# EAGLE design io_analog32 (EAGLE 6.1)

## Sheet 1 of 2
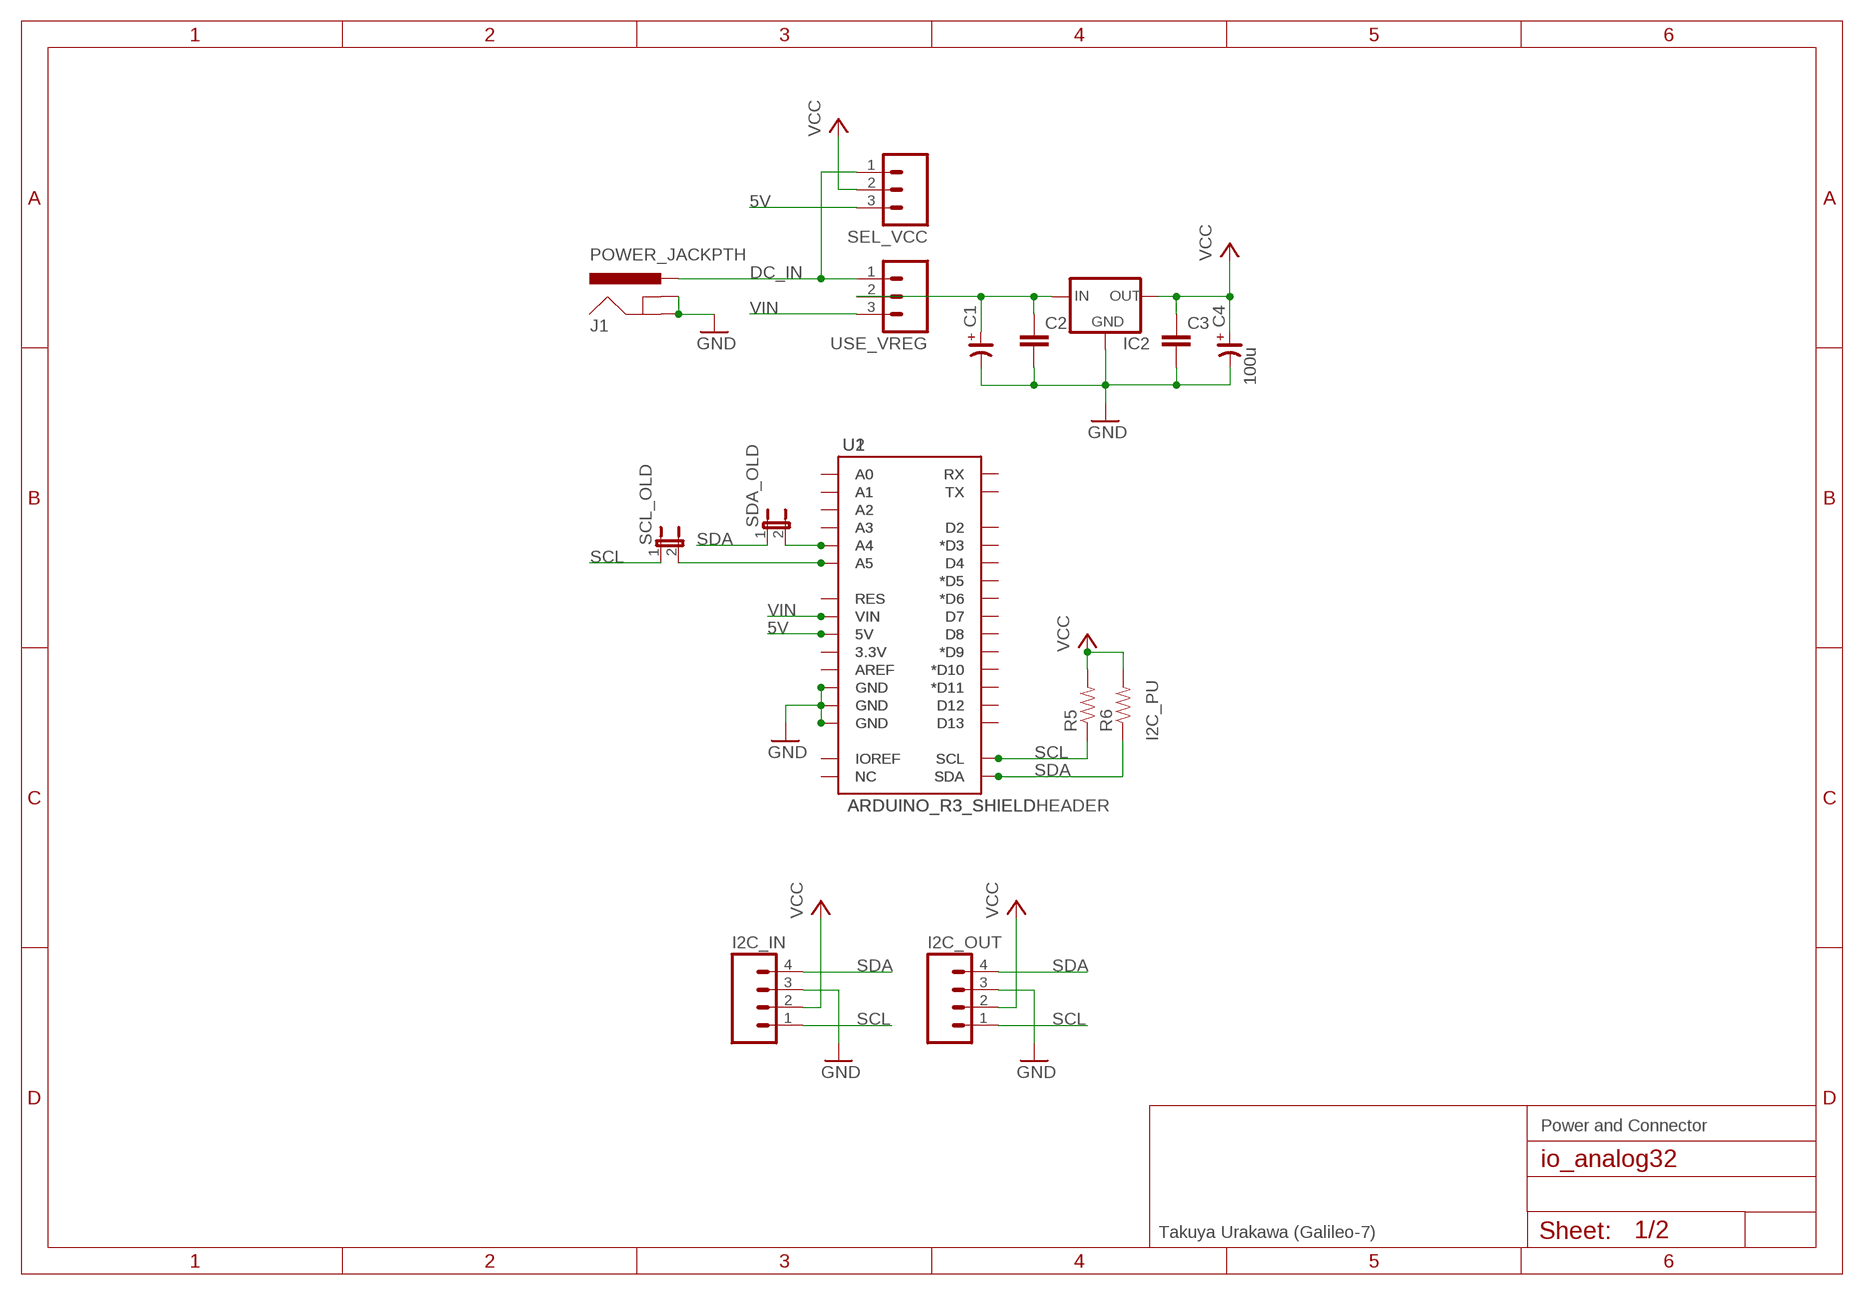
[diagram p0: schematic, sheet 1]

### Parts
C1  CP_E-025X065  [CE-025X065]
C2  CAPPTH1  [CAP-PTH-5MM]
C3  CAPPTH1  [CAP-PTH-5MM]
C4  100u  CP_E-025X065  [CE-025X065]
I2C_IN  M04PTH  [1X04]
I2C_OUT  M04PTH  [1X04]
IC2  V_REG_78XXSINK  [TO220-IGO]
J1  POWER_JACKPTH  [POWER_JACK_PTH]
R5  RESISTORPTH-1/6W  [1/6W-RES]
R6  RESISTORPTH-1/6W  [1/6W-RES]
SCL_OLD  JUMPER-2SMD-NO  [SJ_2S-NO]
SDA_OLD  JUMPER-2SMD-NO  [SJ_2S-NO]
SEL_VCC  M03PTH  [1X03]
U1  ARDUINO_R3_SHIELD  [ARDUINOR3_NOHOLE_NOLABELS]
U2  ARDUINO_R3_SHIELDHEADER  [ARDUINOR3_NODOC]
USE_VREG  M03PTH  [1X03]

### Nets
5V [power]: SEL_VCC.3 U1.5V U2.5V
DC_IN: J1.PWR SEL_VCC.1 USE_VREG.1
GND [power]: C1.- C2.2 C3.2 C4.- I2C_IN.3 I2C_OUT.3 IC2.GND J1.GND J1.GNDBREAK U1.GND@0(GND) U1.GND@2(GND) U2.GND@0(GND) U2.GND@2(GND) ; also sheet 2
N$35: C1.+ C2.1 IC2.IN USE_VREG.2
N$44: U1.RX U2.RX
N$45: U1.TX U2.TX
N$46: U1.D2 U2.D2
N$47: U1.D3(*D3) U2.D3(*D3)
N$48: U1.D4 U2.D4
N$49: U1.D5(*D5) U2.D5(*D5)
N$50: U1.D6(*D6) U2.D6(*D6)
N$51: U1.D7 U2.D7
N$52: U1.D8 U2.D8
N$53: U1.D9(*D9) U2.D9(*D9)
N$54: U1.D10(*D10) U2.D10(*D10)
N$55: U1.D11(*D11) U2.D11(*D11)
N$56: U1.D12 U2.D12
N$57: U1.D13 U2.D13
N$58: U1.A0 U2.A0
N$59: U1.A1 U2.A1
N$60: U1.A2 U2.A2
N$61: U1.A3 U2.A3
N$62: SDA_OLD.2 U1.A4 U2.A4
N$63: SCL_OLD.2 U1.A5 U2.A5
N$65: U1.RES U2.RES
N$67: U1.AREF U2.AREF
N$69: U1.GND@1(GND) U2.GND@1(GND)
N$71: U1.3.3V U2.3.3V
N$74: U1.IOREF U2.IOREF
N$75: U1.NC U2.NC
SCL: I2C_IN.1 I2C_OUT.1 R5.1 SCL_OLD.1 U1.SCL U2.SCL ; also sheet 2
SDA: I2C_IN.4 I2C_OUT.4 R6.1 SDA_OLD.1 U1.SDA U2.SDA ; also sheet 2
VCC [power]: C3.1 C4.+ I2C_IN.2 I2C_OUT.2 IC2.OUT R5.2 R6.2 SEL_VCC.2 ; also sheet 2
VIN [power]: U1.VIN U2.VIN USE_VREG.3

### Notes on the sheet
- I2C_PU
- Power and Connector
- Takuya Urakawa (Galileo-7)

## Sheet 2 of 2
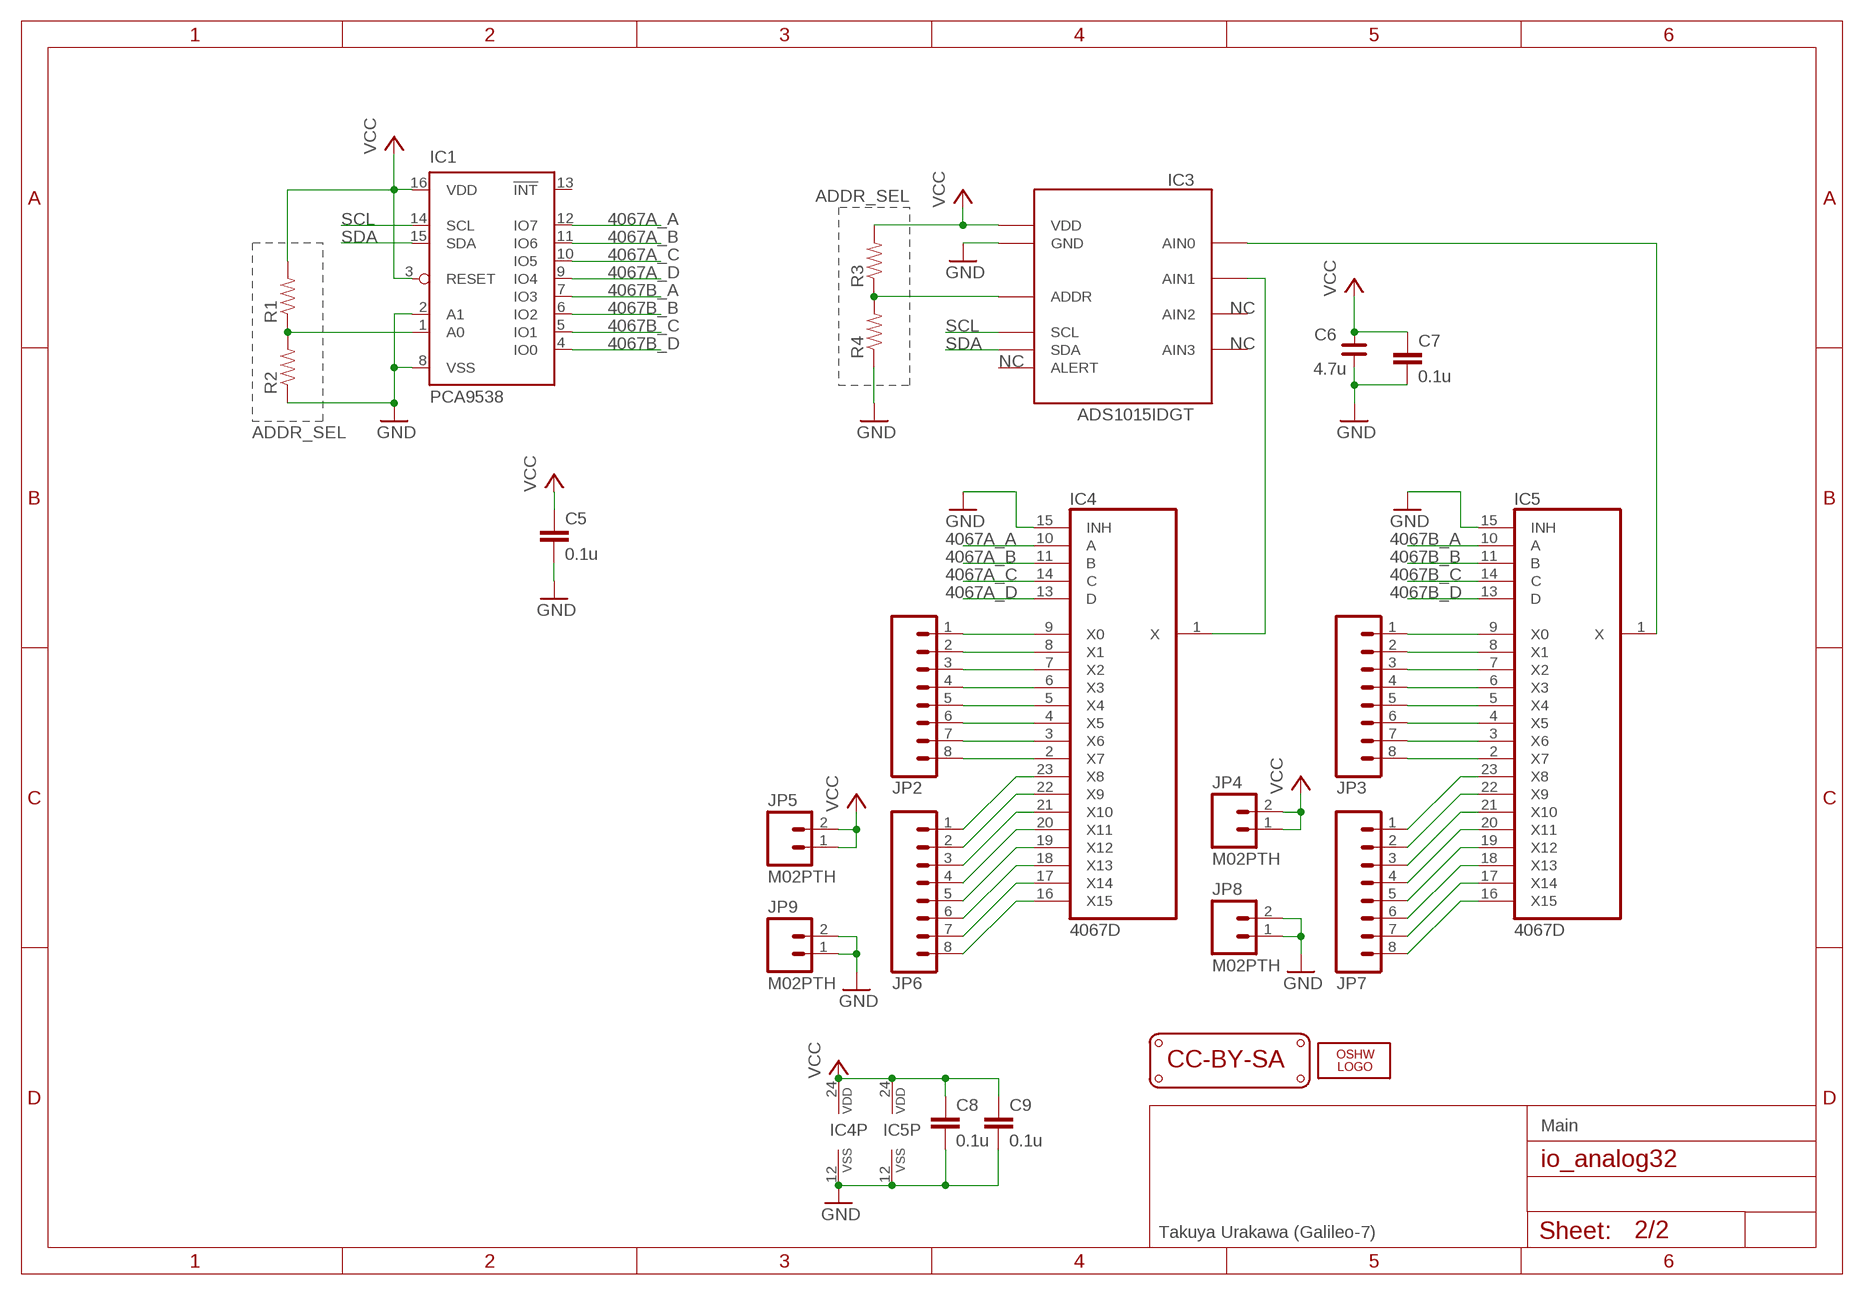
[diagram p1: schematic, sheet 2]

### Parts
C5  0.1u  CAP0805  [0805]
C6  4.7u  C_3216  [C3216]
C7  0.1u  CAP0805  [0805]
C8  0.1u  CAP0805  [0805]
C9  0.1u  CAP0805  [0805]
IC1  PCA9538  [SO16W]
IC3  ADS1015IDGT  [MSOP10_0.5]
IC4  4067D  [SO24W]
IC5  4067D  [SO24W]
JP2  M081X08  [1X08]
JP3  M081X08  [1X08]
JP4  M02PTH  [1X02]
JP5  M02PTH  [1X02]
JP6  M081X08  [1X08]
JP7  M081X08  [1X08]
JP8  M02PTH  [1X02]
JP9  M02PTH  [1X02]
LOGO1  LOGO_CC-BY-SA  [CC-BY-SA]
LOGO2  OSHW_LOGO_FILLX0200-NT  [OSHW_FILLX200_NOTEXT]
R1  RESISTORPTH-1/6W  [1/6W-RES]
R2  RESISTORPTH-1/6W  [1/6W-RES]
R3  RESISTORPTH-1/6W  [1/6W-RES]
R4  RESISTORPTH-1/6W  [1/6W-RES]

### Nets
4067A_A: IC1.12(IO7) IC4.10(A)
4067A_B: IC1.11(IO6) IC4.11(B)
4067A_C: IC1.10(IO5) IC4.14(C)
4067A_D: IC1.9(IO4) IC4.13(D)
4067B_A: IC1.7(IO3) IC5.10(A)
4067B_B: IC1.6(IO2) IC5.11(B)
4067B_C: IC1.5(IO1) IC5.14(C)
4067B_D: IC1.4(IO0) IC5.13(D)
GND [power]: C5.2 C6.1 C7.1 C8.2 C9.2 IC1.2(A1) IC1.8(VSS) IC3.3(GND) IC4.12(VSS) IC4.15(INH) IC5.12(VSS) IC5.15(INH) JP8.1 JP8.2 JP9.1 JP9.2 R2.1 R4.1 ; also sheet 1
N$1: IC5.16(X15) JP7.8
N$2: IC5.17(X14) JP7.7
N$3: IC5.18(X13) JP7.6
N$4: IC5.19(X12) JP7.5
N$5: IC5.20(X11) JP7.4
N$6: IC5.21(X10) JP7.3
N$7: IC5.22(X9) JP7.2
N$8: IC5.23(X8) JP7.1
N$9: IC5.2(X7) JP3.8
N$10: IC5.3(X6) JP3.7
N$11: IC5.4(X5) JP3.6
N$12: IC5.5(X4) JP3.5
N$13: IC5.6(X3) JP3.4
N$14: IC5.7(X2) JP3.3
N$15: IC5.8(X1) JP3.2
N$16: IC5.9(X0) JP3.1
N$17: IC4.16(X15) JP6.8
N$18: IC4.17(X14) JP6.7
N$19: IC4.18(X13) JP6.6
N$20: IC4.19(X12) JP6.5
N$21: IC4.20(X11) JP6.4
N$22: IC4.21(X10) JP6.3
N$23: IC4.22(X9) JP6.2
N$24: IC4.23(X8) JP6.1
N$25: IC4.2(X7) JP2.8
N$26: IC4.3(X6) JP2.7
N$27: IC4.4(X5) JP2.6
N$28: IC4.5(X4) JP2.5
N$29: IC4.6(X3) JP2.4
N$30: IC4.7(X2) JP2.3
N$31: IC4.8(X1) JP2.2
N$32: IC4.9(X0) JP2.1
N$33: IC3.5(AIN1) IC4.1(X)
N$34: IC3.1(ADDR) R3.1 R4.2
N$36: IC3.4(AIN0) IC5.1(X)
N$37: IC1.1(A0) R1.1 R2.2
SCL: IC1.14(SCL) IC3.10(SCL) ; also sheet 1
SDA: IC1.15(SDA) IC3.9(SDA) ; also sheet 1
VCC [power]: C5.1 C6.2 C7.2 C8.1 C9.1 IC1.3(RESET) IC1.16(VDD) IC3.8(VDD) IC4.24(VDD) IC5.24(VDD) JP4.1 JP4.2 JP5.1 JP5.2 R1.2 R3.2 ; also sheet 1
Unconnected: IC1.13(!INT) IC3.2(ALERT) IC3.6(AIN2) IC3.7(AIN3)

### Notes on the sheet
- ADDR_SEL
- NC
- NC
- NC
- ADDR_SEL
- Main
- Takuya Urakawa (Galileo-7)

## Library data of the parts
C1 C4 = rc-master:CP_: POLARIZED CAP
C2 C3 C5 C7-C9 = general:CAP: Capacitor
C6 = rc-master:C_: NON-POLARIZED CAP
I2C_IN I2C_OUT = SparkFun-Connectors:M04: Header 4 Standard 4-pin 0.1" header. Use with straight break away headers (SKU : PRT-00116), right angle break away headers (PRT-00553), swiss pins (PRT-00743), machine pins (PRT-00117), and female headers (PRT-00115). Molex polarized connector foot print use with SKU : PRT-08231 with associated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
IC1 = micro-philips:PCA9538; IC: PCA9538D
IC2 = SparkFun-PowerIC:V_REG_78XX: Voltage Regulator Standard 7805 5V regulator. IGO (Input Ground Output). Spark Fun Electronics SKU : COM-00107
IC3 = bt_adc:ADS1015: Ti ADS1015 12-bit ADC Ultra-Small, Low-Power, 12-Bit Analog-to-Digital Converter with Internal Reference The ADS1013, ADS1014, and ADS1015 are precision analog-to-digital converters (ADCs) with 12 bits of resolution offered in an ultra-small, leadless QFN-10 package or an MSOP-10 package. \ Source: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
IC4 IC5 = 40xx:4067: 16-channel ANALOG MULTIPLEXER
J1 = SparkFun-Connectors:POWER_JACK: Power Jack This is the standard 5.5mm barrel jack for power. The PTH is the most common, proven, reliable, footprint. The Slot footprint only works if the mill layer is transmitted to the PCB fab house so be warned. Spark Fun Electronics SKU : PRT-00119 SMT: CONN-08106 Mating wall wart : TOL-00298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
JP2 JP3 JP6 JP7 = SparkFun-Connectors:M08: Header 8 Standard 8-pin 0.1" header. Use with straight break away headers (SKU : PRT-00116), right angle break away headers (PRT-00553), swiss pins (PRT-00743), machine pins (PRT-00117), and female headers (PRT-00115).
JP4 JP5 JP8 JP9 = SparkFun-Connectors:M02: Standard 2-pin 0.1" header. Use with
LOGO1 = dp_devices:LOGO_CC-BY-SA
LOGO2 = ohw-logo:OSHW_LOGO_FILL
R1-R6 = general:RESISTOR: Resistor
SCL_OLD SDA_OLD = SparkFun-Passives:JUMPER-2: Jumper
SEL_VCC USE_VREG = SparkFun-Connectors:M03: Header 3 Standard 3-pin 0.1" header. Use with straight break away headers (SKU : PRT-00116), right angle break away headers (PRT-00553), swiss pins (PRT-00743), machine pins (PRT-00117), and female headers (PRT-00115). Molex polarized connector foot print use with SKU : PRT-08232 with associated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
U1 = arduino_shield:ARDUINO_R3_SHIELD; U: ArduinoR3
U2 = arduino_shield:ARDUINO_R3_SHIELD

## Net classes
1 power: width 0.305 mm, clearance 0.152 mm

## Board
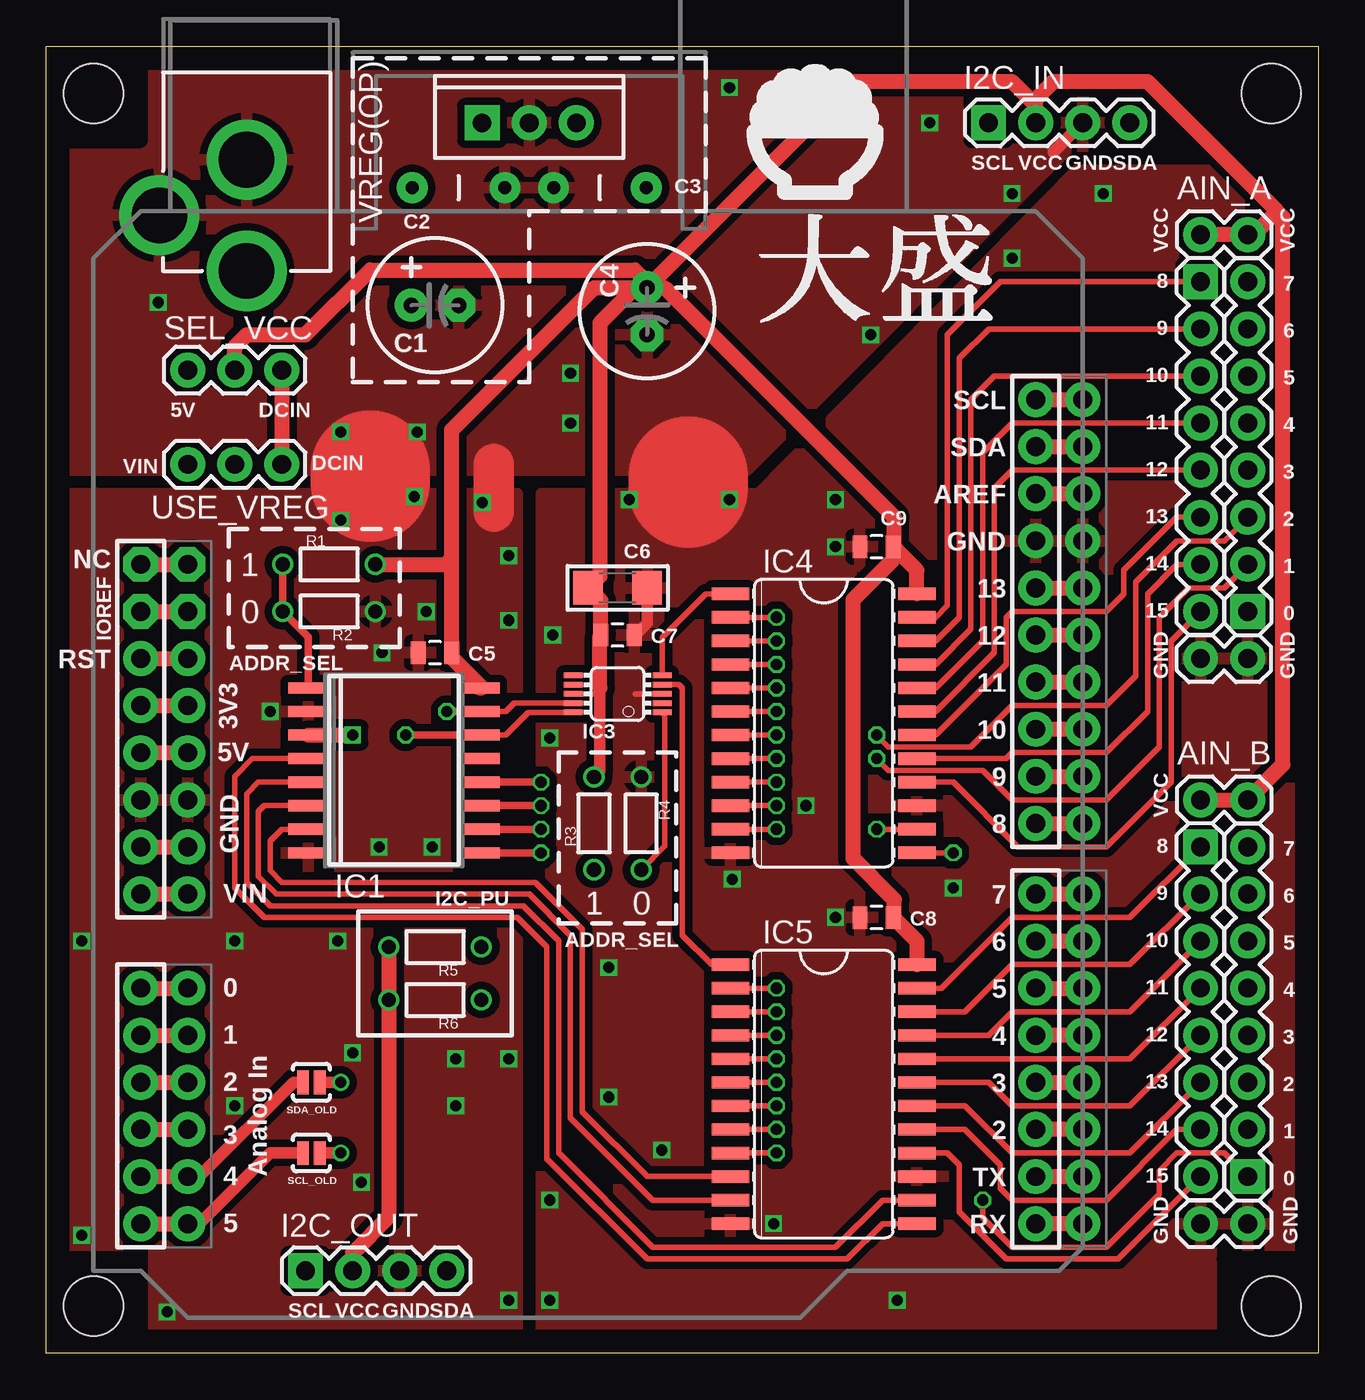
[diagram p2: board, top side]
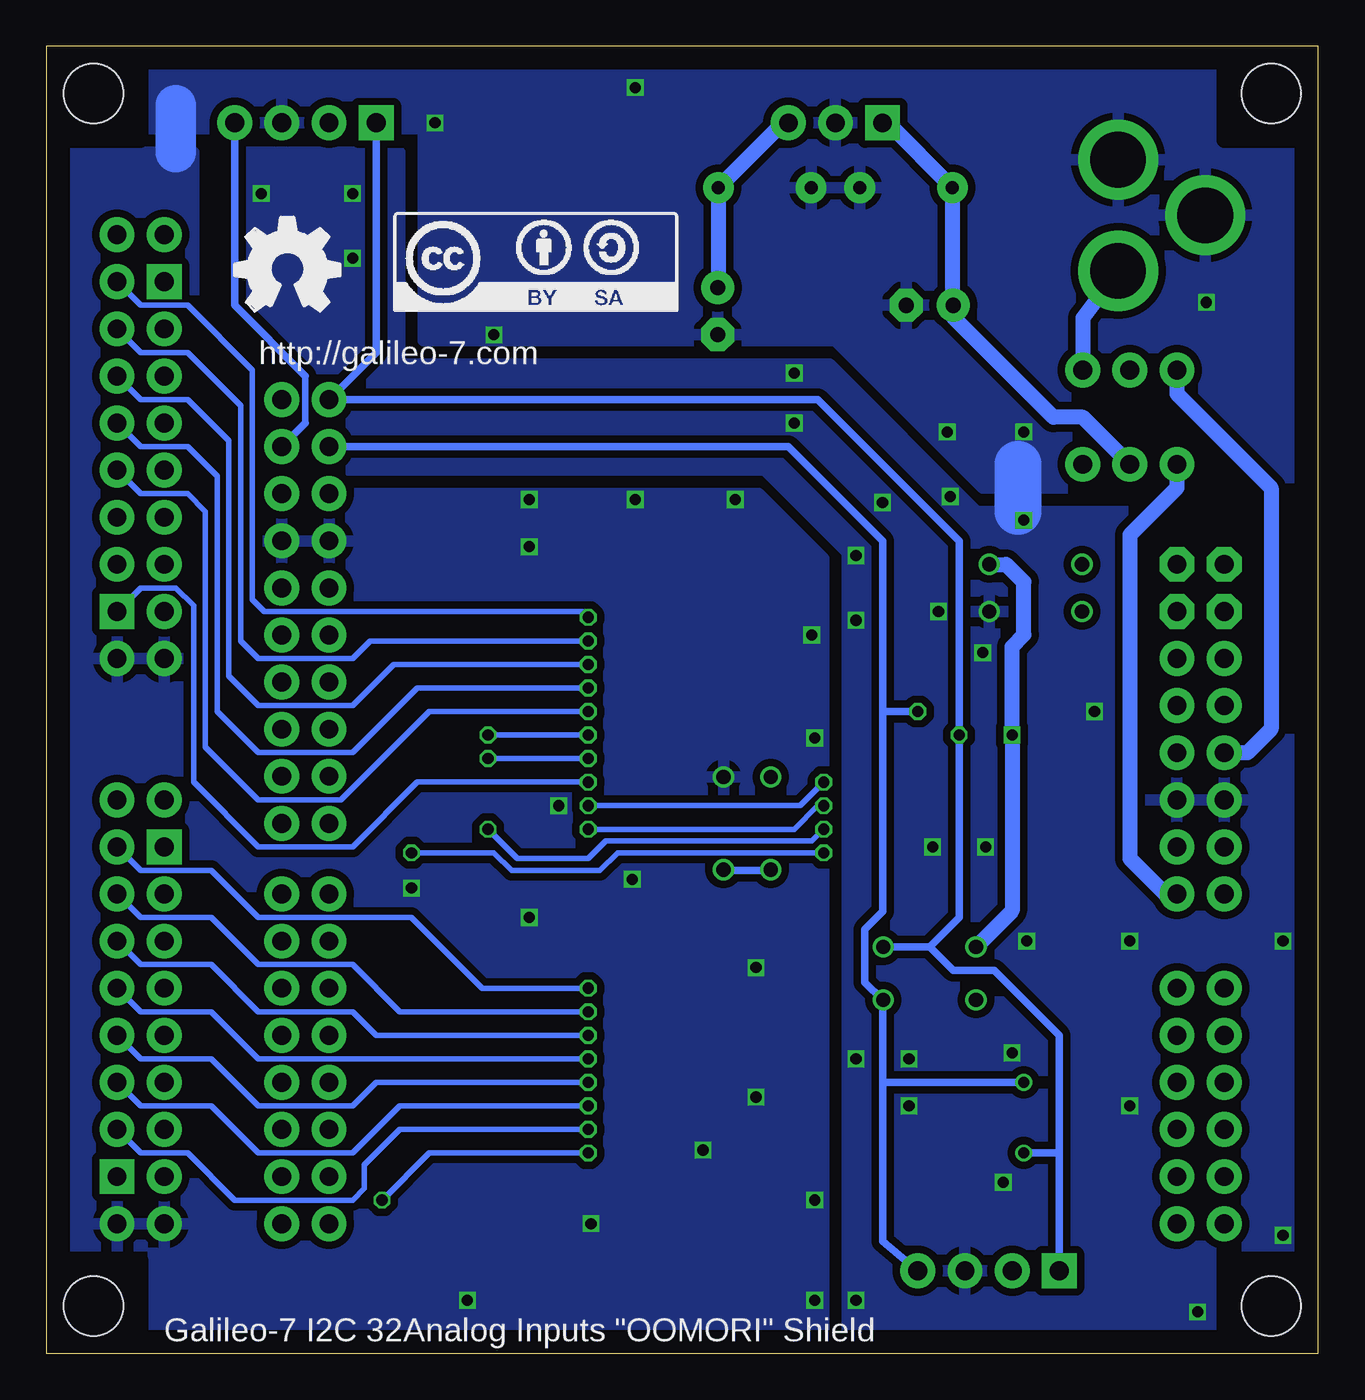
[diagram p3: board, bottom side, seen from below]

Size 68.58 x 70.48 mm. Coordinates in mm from the lower left corner, seen from the top.
Outline: 0,0 0,70.48 68.58,70.48 68.58,0 0,0
Copper layers (1*2*15*16): Top 0.035mm / dielectric 0.2mm / Route2 0.0175mm / dielectric 1.1mm / Route15 0.0175mm / dielectric 0.2mm / Bottom 0.035mm
Design rules: minimum track width 6mil, minimum drill 12mil, track to track 6mil, track to pad 6mil, pad to pad 6mil, via to via 6mil, smd to smd 0mil, copper to edge 50mil, drill to drill 10mil, minimum pad ring 6mil, minimum via ring 6mil, stop-mask expansion 2mil, vias tented up to drill 25mil, thermal gap 15mil
Holes 3.2 mm at 66.04,67.94 66.04,2.54 2.54,2.54 2.54,67.94
tRestrict: area 63.5,65.4 to 68.6,70.5; area 63.5,0 to 68.6,5.1; area 0,0 to 5.1,5.1; area 0,65.4 to 5.1,70.5
bRestrict: area 0,0 to 5.1,5.1; area 63.5,0 to 68.6,5.1; area 63.5,65.4 to 68.6,70.5; area 0,65.4 to 5.1,70.5

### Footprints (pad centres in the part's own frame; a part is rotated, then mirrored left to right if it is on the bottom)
CE-025X065 = drill 0.813 pad 1.778: + -1.27,0 | drill 0.813 pad 1.778 octagon: - 1.27,0
CAP-PTH-5MM = drill 0.7 pad 1.651: 1 -2.5,0; 2 2.5,0
0805 = smd 0.8 x 1.2: 1 -0.9,0; 2 0.9,0
C3216 = smd 1.6 x 1.8: 1 -1.587,0; 2 1.587,0
1X04 = drill 1.016 pad 1.88 square: 1 0,0 | drill 1.016 pad 1.88: 2 2.54,0; 3 5.08,0; 4 7.62,0
SO16W = smd 0.6 x 2.2: 1 -4.445,-4.6; 2 -3.175,-4.6; 3 -1.905,-4.6; 4 -0.635,-4.6; 5 0.635,-4.6; 6 1.905,-4.6; 7 3.175,-4.6; 8 4.445,-4.6; 9 4.445,4.6; 10 3.175,4.6; 11 1.905,4.6; 12 0.635,4.6; 13 -0.635,4.6; 14 -1.905,4.6; 15 -3.175,4.6; 16 -4.445,4.6
TO220-IGO = drill 1 pad 1.88: GND 0,0; OUT 2.54,0 | drill 1 pad 1.88 square: IN -2.54,0
MSOP10_0.5 = smd 0.3 x 1.02: 1 -1,-2.4; 2 -0.5,-2.4; 3 0,-2.4; 4 0.5,-2.4; 5 1,-2.4; 6 1,2.4; 7 0.5,2.4; 8 0,2.4; 9 -0.5,2.4; 10 -1,2.4
SO24W = smd 0.66 x 2.032: 1 -6.985,-5.029; 2 -5.715,-5.029; 3 -4.445,-5.029; 4 -3.175,-5.029; 5 -1.905,-5.029; 6 -0.635,-5.029; 7 0.635,-5.029; 8 1.905,-5.029; 9 3.175,-5.029; 10 4.445,-5.029; 11 5.715,-5.029; 12 6.985,-5.029; 13 6.985,5.029; 14 5.715,5.029; 15 4.445,5.029; 16 3.175,5.029; 17 1.905,5.029; 18 0.635,5.029; 19 -0.635,5.029; 20 -1.905,5.029; 21 -3.175,5.029; 22 -4.445,5.029; 23 -5.715,5.029; 24 -6.985,5.029
POWER_JACK_PTH = drill 2.997 pad 4.318: GND 0,7.7; GNDBREAK 4.7,10.7; PWR 0,13.7
1X08 = drill 1.016 pad 1.88 square: 1 0,0 | drill 1.016 pad 1.88: 2 2.54,0; 3 5.08,0; 4 7.62,0; 5 10.16,0; 6 12.7,0; 7 15.24,0; 8 17.78,0
1X02 = drill 1.016 pad 1.88: 1 0,0; 2 2.54,0
1/6W-RES = drill 0.762: 1 -2.5,0; 2 2.5,0
SJ_2S-NO = smd 0.635 x 1.27: 1 -0.45,0; 2 0.45,0
1X03 = drill 1.016 pad 1.88: 1 0,0; 2 2.54,0; 3 5.08,0
ARDUINOR3_NOHOLE_NOLABELS = drill 1.016 pad 1.88: 3.3V 50.8,26.67; 5V 50.8,29.21; A0 50.8,41.91; A1 50.8,44.45; A2 50.8,46.99; A3 50.8,49.53; A4 50.8,52.07; A5 50.8,54.61; AREF 2.54,15.24; D2 2.54,49.53; D3 2.54,46.99; D4 2.54,44.45; D5 2.54,41.91; D6 2.54,39.37; D7 2.54,36.83; D8 2.54,33.02; D9 2.54,30.48; D10 2.54,27.94; D11 2.54,25.4; D12 2.54,22.86; D13 2.54,20.32; GND@0 50.8,31.75; GND@1 50.8,34.29; GND@2 2.54,17.78; RES 50.8,24.13; RX 2.54,54.61; SCL 2.54,10.16; SDA 2.54,12.7; TX 2.54,52.07; VIN 50.8,36.83 | drill 1.016 pad 1.88 octagon: IOREF 50.8,21.59; NC 50.8,19.05
ARDUINOR3_NODOC = drill 1.016 pad 1.88: 3.3V 50.8,26.67; 5V 50.8,29.21; A0 50.8,41.91; A1 50.8,44.45; A2 50.8,46.99; A3 50.8,49.53; A4 50.8,52.07; A5 50.8,54.61; AREF 2.54,15.24; D2 2.54,49.53; D3 2.54,46.99; D4 2.54,44.45; D5 2.54,41.91; D6 2.54,39.37; D7 2.54,36.83; D8 2.54,33.02; D9 2.54,30.48; D10 2.54,27.94; D11 2.54,25.4; D12 2.54,22.86; D13 2.54,20.32; GND@0 50.8,31.75; GND@1 50.8,34.29; GND@2 2.54,17.78; RES 50.8,24.13; RX 2.54,54.61; SCL 2.54,10.16; SDA 2.54,12.7; TX 2.54,52.07; VIN 50.8,36.83 | drill 1.016 pad 1.88 octagon: IOREF 50.8,21.59; NC 50.8,19.05

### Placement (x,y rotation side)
C1  20.95,56.52 0 top
C2  22.23,62.87 0 top
C3  29.84,62.87 180 top
C4  32.38,56.2 270 top
C5  20.95,37.78 180 top
C6  30.8,41.27 180 top
C7  30.8,38.73 180 top
C8  44.77,23.5 180 top
C9  44.77,43.5 180 top
I2C_IN  50.8,66.36 0 top
I2C_OUT  13.97,4.45 0 top
IC1  18.73,31.43 270 top
IC2  26.04,66.36 0 top
IC3  30.8,35.56 90 top
IC4  41.91,33.97 270 top
IC5  41.91,13.97 270 top
J1  10.79,72.07 180 top
JP2  64.77,40.01 90 top
JP3  64.77,9.53 90 top
JP4  62.23,29.84 0 top
JP5  62.23,60.33 0 top
JP6  62.23,57.78 270 top
JP7  62.23,27.3 270 top
JP8  62.23,6.99 0 top
JP9  64.77,37.47 180 top
LOGO1  49.85,56.2 0 bottom
LOGO2  58.42,56.2 0 bottom
R1  15.24,42.55 0 top
R2  15.24,40.01 180 top
R3  29.53,28.57 90 top
R4  32.07,28.57 270 top
R5  20.95,21.91 180 top
R6  20.95,19.05 180 top
SCL_OLD  14.29,10.79 180 top
SDA_OLD  14.29,14.61 180 top
SEL_VCC  12.7,53.02 180 top
U1  55.88,61.59 180 top
U2  58.42,61.59 180 top
U$1  [OMORI_LOGO]  37.78,62.23 0 top
U$2  [OMORI_LOGO2]  38.42,55.56 0 top
USE_VREG  12.7,47.94 180 top

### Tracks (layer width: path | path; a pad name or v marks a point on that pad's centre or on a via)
5V
  Top 0.813: U1.5V U2.5V
  Bottom 0.813: U1.5V 3.81,32.38 2.54,33.66 2.54,46.67 7.62,51.75 SEL_VCC.3
4067A_A  (via drill 0.6)
  Top 0.305: v39.37,29.53 IC4.10
  Top 0.406: IC1.12 v26.67,30.8
  Bottom 0.305: v26.67,30.8 27.94,29.53 v39.37,29.53
4067A_B  (via drill 0.6)
  Top 0.305: v39.37,28.26 IC4.11
  Top 0.406: IC1.11 v26.67,29.53
  Bottom 0.305: v26.67,29.53 26.99,29.53 28.26,28.26 v39.37,28.26
4067A_C  (via drill 0.6)
  Top 0.305: v44.77,28.26 IC4.14
  Top 0.406: IC1.10 v26.67,28.26
  Bottom 0.305: v26.67,28.26 27.3,27.62 38.42,27.62 39.37,26.67 43.18,26.67 v44.77,28.26
4067A_D  (via drill 0.6)
  Top 0.305: IC4.13 v48.9,26.99
  Top 0.406: IC1.9 v26.67,26.99
  Bottom 0.305: v48.9,26.99 44.45,26.99 43.5,26.04 38.73,26.04 37.78,26.99 v26.67,26.99
4067B_A
  Top 0.305: IC1.7 12.7,28.26 12.06,27.62 12.06,26.04 12.7,25.4 26.35,25.4 28.89,22.86 28.89,13.02 32.38,9.53 IC5.10
4067B_B
  Top 0.305: IC1.6 11.75,29.53 11.43,29.21 11.43,25.72 12.38,24.77 26.04,24.77 28.26,22.54 28.26,12.7 32.7,8.26 IC5.11
4067B_C
  Top 0.305: IC1.5 11.43,30.8 10.79,30.16 10.79,25.4 12.06,24.13 25.72,24.13 27.62,22.23 27.62,10.79 32.7,5.71 42.55,5.71 45.09,8.26 IC5.14
4067B_D
  Top 0.305: IC1.4 11.11,32.07 10.16,31.11 10.16,25.08 11.75,23.5 25.4,23.5 26.99,21.91 26.99,10.48 32.38,5.08 43.18,5.08 45.09,6.99 IC5.13
  Top 0.406: IC5.13 46.99,6.99
DC_IN
  Top 0.813: SEL_VCC.1 USE_VREG.1
  Bottom 0.813: J1.PWR 12.7,55.83 SEL_VCC.1
GND  (via drill 0.6)
  Top 0.305: IC3.3 31.75,35.56
  Top 0.61: C6.1 32.38,39.37 31.75,38.73 C7.1 | I2C_IN.3 54.29,64.77 | v31.43,46.04 34.61,46.04 34.61,46.67 | 17.14,44.61 17.46,44.93
  Top 0.813: 17.46,48.74 17.46,48.58
  Top 1.016: 17.46,46.99 17.46,44.93
  Top 2.184: 24.13,45.4 24.13,47.94
  Top 6.452: 17.46,47.62 17.46,46.99 | 34.61,47.31 34.61,46.67
  Bottom 2.184: 61.59,67.31 61.59,64.77
  Bottom 2.54: 16.19,47.94 16.19,45.4
  other vias: 36.99,25.56 40.96,29.53 42.55,23.5 48.9,25.08 42.55,43.5 17.94,27.3 42.55,46.04 20.8,27.3 18.1,37.78 20.48,40.01 23.5,45.88 24.92,39.53 22.07,15.88 22.07,13.34 24.92,15.88 27.15,2.86 45.88,2.86 24.92,2.86 6.51,2.22 1.91,6.35 15.72,22.23 12.06,34.61 10.16,22.23 27.3,38.73 56.99,62.55 20,49.69 6.03,56.67 15.88,49.69 36.83,68.26 44.45,54.93 30.32,13.81 33.18,10.95 30.32,20.8 27.15,33.18 47.62,66.36 16.51,16.19 1.91,22.23 15.88,44.93 36.83,46.04 19.84,46.2 28.26,52.86 28.26,50.16 24.92,43.02 39.21,6.99 27.15,8.26 16.99,9.21 52.07,62.55 10.16,13.34 52.07,59.05
  pour Top (isolate 0.406): 26.67,46.35 38.42,46.35 55.56,63.82 68.58,63.82 68.58,0 26.67,0
  pour Top (isolate 0.406): 0,46.35 25.4,46.35 25.4,0 0,0
  pour Bottom (isolate 0.406): 49.53,64.77 59.69,64.77 59.69,47.62 29.84,47.62 25.4,43.18 25.4,0 0,0 0,45.4 18.41,45.4 26.35,53.34 49.53,53.34
  pour Bottom (isolate 0.406): 30.16,46.35 26.67,42.86 26.67,0 68.58,0 68.58,64.77 60.64,64.77 60.64,46.35
  pour Top (isolate 0.406): 0,47.62 37.78,47.62 55.24,65.09 68.58,65.09 68.58,70.48 0,70.48
  pour Bottom (isolate 0.406): 18.1,46.67 26.04,54.61 48.26,54.61 48.26,66.04 68.58,66.04 68.58,70.48 0,70.48 0,46.67
N$1
  Top 0.305: IC5.16 48.58,10.79 49.21,10.16 49.21,7.62 51.75,5.08 57.78,5.08 JP7.8
N$2
  Top 0.305: IC5.17 49.53,12.06 51.44,10.16 51.44,8.89 52.07,8.26 57.15,8.26 60.96,12.06 JP7.7
N$3
  Top 0.305: IC5.18 49.53,13.34 52.07,10.79 58.42,10.79 JP7.6
N$4
  Top 0.305: IC5.19 50.8,14.61 52.07,13.34 58.42,13.34 JP7.5
N$5
  Top 0.305: IC5.20 58.42,15.88 JP7.4
N$6
  Top 0.305: IC5.21 50.8,17.14 52.07,18.41 58.42,18.41 JP7.3
N$7
  Top 0.305: IC5.22 49.53,18.41 52.07,20.95 58.42,20.95 JP7.2
N$8
  Top 0.305: IC5.23 48.26,19.68 52.07,23.5 58.42,23.5 JP7.1
N$9  (via drill 0.6)
  Top 0.305: v39.37,19.68 IC5.2
  Bottom 0.305: JP3.8 63.5,26.04 59.69,26.04 57.15,23.5 48.9,23.5 45.09,19.68 v39.37,19.68
N$10  (via drill 0.6)
  Top 0.305: IC5.3 v39.37,18.41
  Bottom 0.305: v39.37,18.41 49.53,18.41 52.07,20.95 57.15,20.95 59.69,23.5 63.5,23.5 JP3.7
N$11  (via drill 0.6)
  Top 0.305: v39.37,17.14 IC5.4
  Bottom 0.305: JP3.6 63.5,20.95 59.69,20.95 57.15,18.41 52.07,18.41 50.8,17.14 v39.37,17.14
N$12  (via drill 0.6)
  Top 0.305: IC5.5 v39.37,15.88
  Bottom 0.305: v39.37,15.88 57.15,15.88 59.69,18.41 63.5,18.41 JP3.5
N$13  (via drill 0.6)
  Top 0.305: IC5.6 v39.37,14.61
  Bottom 0.305: JP3.4 63.5,15.88 59.69,15.88 57.15,13.34 52.07,13.34 50.8,14.61 v39.37,14.61
N$14  (via drill 0.6)
  Top 0.305: IC5.7 v39.37,13.34
  Bottom 0.305: v39.37,13.34 49.53,13.34 52.07,10.79 57.15,10.79 59.69,13.34 63.5,13.34 JP3.3
N$15  (via drill 0.6)
  Top 0.305: IC5.8 v39.37,12.06
  Bottom 0.305: v39.37,12.06 49.53,12.06 51.44,10.16 51.44,8.89 52.07,8.26 58.42,8.26 60.96,10.79 63.5,10.79 JP3.2
N$16  (via drill 0.6)
  Top 0.305: JP3.1 63.5,10.79 60.96,10.79 60.01,9.84 60.01,8.57 57.15,5.71 52.07,5.71 50.48,7.3 v50.48,8.26 | IC5.9 v39.37,10.79
  Bottom 0.305: v39.37,10.79 47.94,10.79 v50.48,8.26
N$17
  Top 0.305: IC4.16 48.9,30.8 52.39,27.3 57.15,27.3 60.64,30.8 60.64,38.42 JP6.8
N$18
  Top 0.305: IC4.17 51.75,32.07 52.07,32.38 57.15,32.38 59.37,34.61 59.37,40.96 60.96,42.55 JP6.7
N$19
  Top 0.305: IC4.18 47.94,33.34 51.75,37.15 51.75,39.69 52.07,40.01 57.15,40.01 58.1,40.96 58.1,42.23 60.96,45.09 JP6.6
N$20
  Top 0.305: IC4.19 47.94,34.61 51.12,37.78 51.12,46.67 52.07,47.62 JP6.5
N$21
  Top 0.305: IC4.20 47.94,35.88 50.48,38.42 50.48,48.58 52.07,50.16 JP6.4
N$22
  Top 0.305: IC4.21 47.94,37.15 49.85,39.05 49.85,51.44 51.12,52.7 JP6.3
N$23
  Top 0.305: IC4.22 47.94,38.42 49.21,39.69 49.21,53.66 50.8,55.24 JP6.2
N$24
  Top 0.305: IC4.23 47.94,39.69 48.58,40.32 48.58,54.93 51.44,57.78 JP6.1
N$25  (via drill 0.6)
  Top 0.305: v39.37,39.69 IC4.2
  Bottom 0.305: JP2.8 63.5,56.52 60.96,56.52 57.47,53.02 57.47,40.64 56.83,40.01 39.69,40.01 v39.37,39.69
N$26  (via drill 0.6)
  Top 0.305: v39.37,38.42 IC4.3
  Bottom 0.305: JP2.7 63.5,53.98 60.96,53.98 58.1,51.12 58.1,38.42 57.15,37.47 52.07,37.47 51.12,38.42 v39.37,38.42
N$27  (via drill 0.6)
  Top 0.305: v39.37,37.15 IC4.4 37.47,37.15
  Bottom 0.305: JP2.6 63.5,51.44 60.96,51.44 58.74,49.21 58.74,36.51 57.15,34.92 52.07,34.92 49.85,37.15 v39.37,37.15
N$28  (via drill 0.6)
  Top 0.305: IC4.5 v39.37,35.88
  Bottom 0.305: v39.37,35.88 48.58,35.88 52.07,32.38 57.15,32.38 59.37,34.61 59.37,47.31 60.96,48.9 63.5,48.9 JP2.5
N$29  (via drill 0.6)
  Top 0.305: IC4.6 v39.37,34.61
  Bottom 0.305: v39.37,34.61 47.94,34.61 52.7,29.84 57.15,29.84 60.01,32.7 60.01,45.4 60.96,46.35 63.5,46.35 JP2.4
N$30  (via drill 0.6)
  Top 0.305: JP2.3 63.5,43.81 60.96,43.81 58.74,41.59 58.74,36.51 57.15,34.92 52.07,34.92 49.85,32.7 45.4,32.7 v44.77,33.34 | IC4.7 v39.37,33.34
  Bottom 0.305: v39.37,33.34 v44.77,33.34
N$31  (via drill 0.6)
  Top 0.305: JP2.2 63.5,41.27 61.59,41.27 60.01,39.69 60.01,32.7 57.15,29.84 52.07,29.84 50.48,31.43 45.4,31.43 v44.77,32.07 | IC4.8 v39.37,32.07
  Bottom 0.305: v39.37,32.07 v44.77,32.07
N$32  (via drill 0.6)
  Top 0.305: IC4.9 v39.37,30.8
  Bottom 0.305: v39.37,30.8 48.58,30.8 52.07,27.3 57.15,27.3 60.64,30.8 60.64,40.32 61.59,41.27 63.5,41.27 JP2.1
N$33
  Top 0.305: IC3.5 33.2,38.59 35.56,40.96 IC4.1
N$34
  Top 0.305: 32.03,26.04 R4.2 33.34,27.34 33.34,34.42 IC3.1
  Bottom 0.406: R4.2 32.07,26.04 29.53,26.04 R3.1
N$35
  Bottom 0.813: IC2.IN 23.22,66.36 C2.1 19.73,56.55 C1.+ 19.68,55.88 14.29,50.48 12.7,50.48 USE_VREG.2
N$36
  Top 0.305: IC3.4 34.11,36.06 34.29,35.88 34.29,22.54 35.88,20.95 IC5.1
N$37
  Top 0.406: IC1.1 14.13,38.61 R2.2 R1.1
N$44
  Top 0.813: U2.RX U1.RX
N$45
  Top 0.813: U1.TX U2.TX
N$46
  Top 0.813: U2.D2 U1.D2
N$47
  Top 0.813: U1.D3 U2.D3
N$48
  Top 0.813: U2.D4 U1.D4
N$49
  Top 0.813: U1.D5 U2.D5
N$50
  Top 0.813: U1.D6 U2.D6
N$51
  Top 0.813: U1.D7 U2.D7
N$52
  Top 0.813: U1.D8 U2.D8
N$53
  Top 0.813: U1.D9 U2.D9
N$54
  Top 0.813: U1.D10 U2.D10
N$55
  Top 0.813: U1.D11 U2.D11
N$56
  Top 0.813: U1.D12 U2.D12
N$57
  Top 0.813: U1.D13 U2.D13
N$58
  Top 0.813: U1.A0 U2.A0
N$59
  Top 0.813: U1.A1 U2.A1
N$60
  Top 0.813: U1.A2 U2.A2
N$61
  Top 0.813: U1.A3 U2.A3
N$62
  Top 0.61: U2.A4 8.26,9.53 13.34,14.61 SDA_OLD.2
  Top 0.813: U1.A4 U2.A4
N$63
  Top 0.61: U2.A5 8.26,6.99 12.06,10.79 SCL_OLD.2
  Top 0.813: U1.A5 U2.A5
N$65
  Top 0.813: U1.RES U2.RES
N$67
  Top 0.813: U1.AREF U2.AREF
N$69
  Top 0.813: U1.GND@1 U2.GND@1
N$71
  Top 0.813: U1.3.3V U2.3.3V
N$74
  Top 0.813: U1.IOREF U2.IOREF
N$75
  Top 0.813: U1.NC U2.NC
SCL  (via drill 0.6)
  Top 0.305: IC3.10 25.99,34.56 24.77,33.34 IC1.14
  Top 0.406: IC1.14 v19.37,33.34
  Top 0.61: SCL_OLD.1 v15.88,10.79
  Top 0.813: U1.SCL U2.SCL
  Bottom 0.406: I2C_IN.1 50.8,53.98 U1.SCL 26.99,51.44 19.37,43.81 v19.37,33.34 19.37,23.5 20.95,21.91 | R5.1 20.95,21.91 | 13.97,10.79 13.97,17.14 17.46,20.64 19.68,20.64 20.95,21.91 | I2C_OUT.1 13.97,10.79 | 13.97,10.79 v15.88,10.79
SDA  (via drill 0.6)
  Top 0.305: IC3.9 25.22,35.06 24.77,34.61 IC1.15
  Top 0.406: IC1.15 v21.59,34.61
  Top 0.61: SDA_OLD.1 v15.88,14.61
  Top 0.813: U1.SDA U2.SDA
  Bottom 0.356: 54.61,50.16 54.61,52.7
  Bottom 0.406: U1.SDA 28.57,48.9 23.5,43.81 23.5,34.61 | v21.59,34.61 23.5,34.61 | U2.SDA 54.61,50.16 | 54.61,52.7 58.42,56.52 I2C_IN.4 | 23.5,34.61 23.5,23.81 24.45,22.86 24.45,20 23.5,19.05 | 23.5,19.05 R6.1 23.5,19.01 | v15.88,14.61 23.5,14.61 | 23.5,14.61 23.5,6.03 I2C_OUT.4 | 23.5,19.01 23.5,19.05 | 23.5,19.01 23.5,14.61
VCC  (via drill 0.6)
  Top 0.305: IC3.8 29.53,35.56 29.84,35.88
  Top 0.61: R3.2 29.84,31.39 29.84,35.88 | 21.86,37.52 21.86,40.91 21.91,40.96
  Top 0.813: 29.84,35.88 29.84,38.68 C7.2 29.9,40.59 C6.2 29.84,41.91 29.84,55.56 31.75,57.47 C4.+ | C9.1 45.72,43.55 45.72,45.09 33.34,57.47 C4.+ | IC4.24 46.94,42.23 C9.1 | C4.+ 29.53,57.47 21.86,49.8 21.86,42.86 | IC5.24 46.94,22.22 C8.1 45.72,23.55 45.72,24.45 43.5,26.67 43.5,40.64 45.67,42.81 C9.1 | IC1.16 23.5,35.88 21.86,37.52 C5.1 21.86,42.86 | R1.2 21.54,42.55 21.86,42.86 | JP4.1 JP4.2 66.67,31.75 66.67,61.28 66.36,61.59 | JP5.1 JP5.2 65.09,60.33 66.36,61.59 | IC1.3 v16.51,33.34 | R5.2 R6.2 18.45,7.34 16.51,5.4 I2C_OUT.2 | 66.36,61.59 59.37,68.58 54.29,68.58 53.34,67.63 I2C_IN.2 53.34,67.31 52.07,68.58 43.5,68.58 C4.+ | SEL_VCC.2 10.16,54.29 10.79,54.93 13.97,54.93 17.46,58.42 31.75,58.42 32.38,57.78 C4.+
  Bottom 0.813: C4.+ 32.34,57.51 C3.1 28.85,66.36 IC2.OUT | R6.2 18.41,19.05 | R5.2 16.51,23.85 v16.51,33.34 16.51,38.1 15.88,38.73 15.88,41.59 16.83,42.55 R1.2
VIN
  Top 0.813: U1.VIN U2.VIN
  Bottom 0.813: USE_VREG.3 7.62,46.67 10.16,44.13 10.16,26.67 8.26,24.77 U2.VIN

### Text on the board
tPlace: SCL | VCC | GND | SDA | AIN_A | VREG(OP) | VCC | VCC | 8 | 7 | 9 | 6 | 10 | SCL | 5 | 11 | 5V | DCIN | 4 | SDA | VIN | DCIN | 12 | AREF | 3 | 13 | 2 | GND | NC | 14 | 1 | 13 | 1 | 15 | 0 | 0 | 12 | IOREF | RST | ADDR_SEL | 11 | GND | GND | 3V3 | 10 | 5V | 9 | AIN_B | GND | 8 | VCC | 8 | 7 | 7 | 9 | VIN | I2C_PU | 1 | 0 | 6 | 6 | 10 | ADDR_SEL | 5 | 5 | 11 | 0 | 4 | 4 | 12 | 1 | 3 | 3 | 13 | 2 | 2 | 2 | 14 | 1 | 3 | Analog In | TX | 15 | 4 | 0 | 5 | RX | GND | GND | SCL | VCC | GND | SDA
bPlace: http://galileo-7.com | Galileo-7 I2C 32Analog Inputs "OOMORI" Shield

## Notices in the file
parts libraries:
SparkFun-Connectors: Licensing: CC v3.0 Share-Alike You are welcome to use this library for commercial purposes.
rc-master: Copyright (C) 2007, Bob Starr
